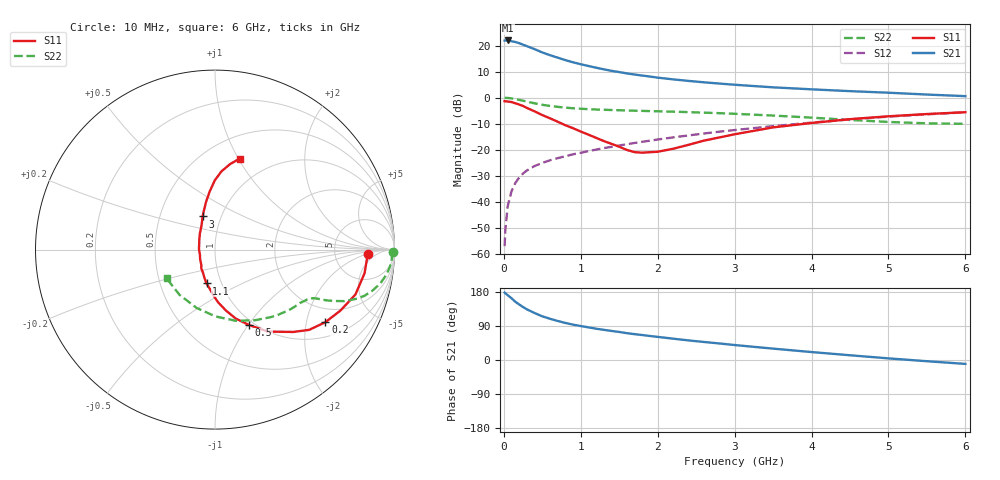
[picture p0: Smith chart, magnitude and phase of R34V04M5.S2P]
! SIEMENS Small Signal Semiconductors
! BFR181
! Si NPN RF Bipolar Junction Transistor in SOT23
! VCE = 4 V  IC = 4.5 mA
! Common Emitter S-Parameters:  May  1996
# GHz  S  MA  R  50
!  f  S11  S21  S12  S22
! GHz  MAG  ANG  MAG  ANG  MAG  ANG  MAG  ANG
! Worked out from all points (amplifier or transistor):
!   36 points, 10 MHz to 6 GHz, reference 50 ohm
!   highest |S21| = 22.0 dB at 50 MHz (marker M1)
!   |S21| within 3 dB of that: start of sweep to 370.3 MHz
!   unconditionally stable (mu >= 1): 1.183 GHz to 3.023 GHz
!   at 250 MHz: K = 0.39, MSG = 24.7 dB, |S12| = -29.1 dB
!   at 1.4 GHz: K = 1.04, MAG = 13.4 dB, |S12| = -18.9 dB
!   at 6 GHz: K = 0.86, MSG = 3.1 dB, |S12| = -5.7 dB
!   S11 on the Smith chart (normalised r, x): 10 MHz: 12, -2; 200 MHz: 1.47, -2.60; 500 MHz: 0.95, -1.01; 1.1 GHz: 0.85, -0.33; 3 GHz: 0.82, +0.31; 6 GHz: 0.72, +1.01
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0.01  0.8533 -1.8  12.47 178.0  0.0014 81.9  0.9933 -0.9
0.02  0.8485 -3.4  12.49 176.1  0.0029 85.7  0.9867 -1.7
0.05  0.8436 -9.0  12.53 171.0  0.0082 84.9  0.9862 -4.2
0.1  0.8216 -17.7  12.1 162.8  0.016 80.5  0.9665 -8.2
0.15  0.7773 -25.9  11.7 153.6  0.023 76.3  0.939 -11.7
0.2  0.7362 -33.3  11.1 146.5  0.0292 73.1  0.9054 -14.7
0.25  0.6896 -40.4  10.38 139.8  0.0349 69.7  0.8711 -17.2
0.3  0.6336 -46.4  9.732 133.6  0.0399 68.0  0.8385 -19.0
0.4  0.5442 -57.1  8.532 123.9  0.0485 64.9  0.7766 -21.7
0.5  0.4619 -65.6  7.374 115.3  0.0556 63.3  0.727 -23.2
0.6  0.4009 -73.3  6.537 108.8  0.0626 62.5  0.6925 -24.2
0.8  0.2945 -86.6  5.253 97.8  0.0748 61.9  0.6418 -25.4
0.9  0.2583 -91.5  4.768 93.3  0.0816 62.4  0.6248 -25.8
1.1  0.1942 -104.1  4.05 86.1  0.0938 63.1  0.6001 -27.0
1.3  0.1464 -116.9  3.491 79.6  0.1071 63.2  0.584 -28.4
1.6  0.0987 -147.1  2.917 70.8  0.1273 63.2  0.5664 -31.0
2.2  0.104 147.2  2.24 56.3  0.172 62.1  0.537 -38.0
3  0.1975 110.6  1.767 39.5  0.2382 57.8  0.4889 -50.2
3.5  0.2681 100.9  1.575 30.0  0.2831 54.0  0.4519 -60.6
4.5  0.3855 90.2  1.331 12.5  0.3813 44.0  0.3723 -89.6
5.5  0.4838 80.0  1.145 -3.2  0.4775 31.5  0.3204 -128.0
6  0.5245 74.9  1.067 -10.3  0.5217 24.4  0.3138 -149.3
